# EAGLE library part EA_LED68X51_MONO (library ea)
ELECRONIC ASSEMBLY GmbH EA LED68x51-A EA LED68x51-B EA LED68x51-G EA LED68x51-R EA LED68x51-W
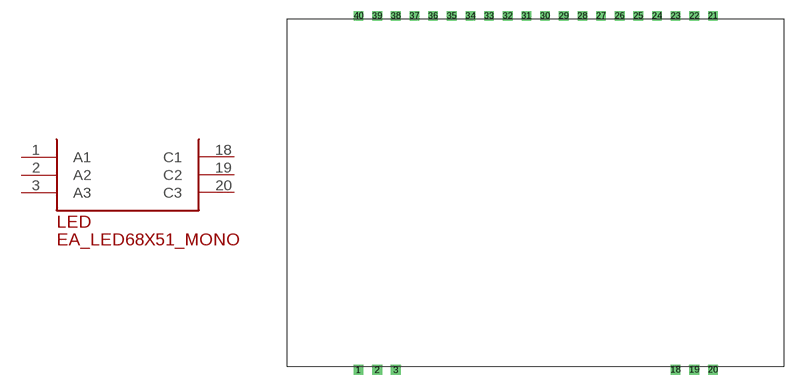
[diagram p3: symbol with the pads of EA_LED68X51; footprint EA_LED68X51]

Designator prefix LED

## EA_LED68X51_MONO  [EA_LED68X51]
1  A1  pas
2  A2  pas
3  A3  pas
18  C1  pas
19  C2  pas
20  C3  pas

## Footprint EA_LED68X51 (pad centres in mm)
drill 0.813 square: 1 0,0; 2 2.54,0; 3 5.08,0; 18 43.18,0; 19 45.72,0; 20 48.26,0; 21 48.26,48.26; 22 45.72,48.26; 23 43.18,48.26; 24 40.64,48.26; 25 38.1,48.26; 26 35.56,48.26; 27 33.02,48.26; 28 30.48,48.26; 29 27.94,48.26; 30 25.4,48.26; 31 22.86,48.26; 32 20.32,48.26; 33 17.78,48.26; 34 15.24,48.26; 35 12.7,48.26; 36 10.16,48.26; 37 7.62,48.26; 38 5.08,48.26; 39 2.54,48.26; 40 0,48.26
